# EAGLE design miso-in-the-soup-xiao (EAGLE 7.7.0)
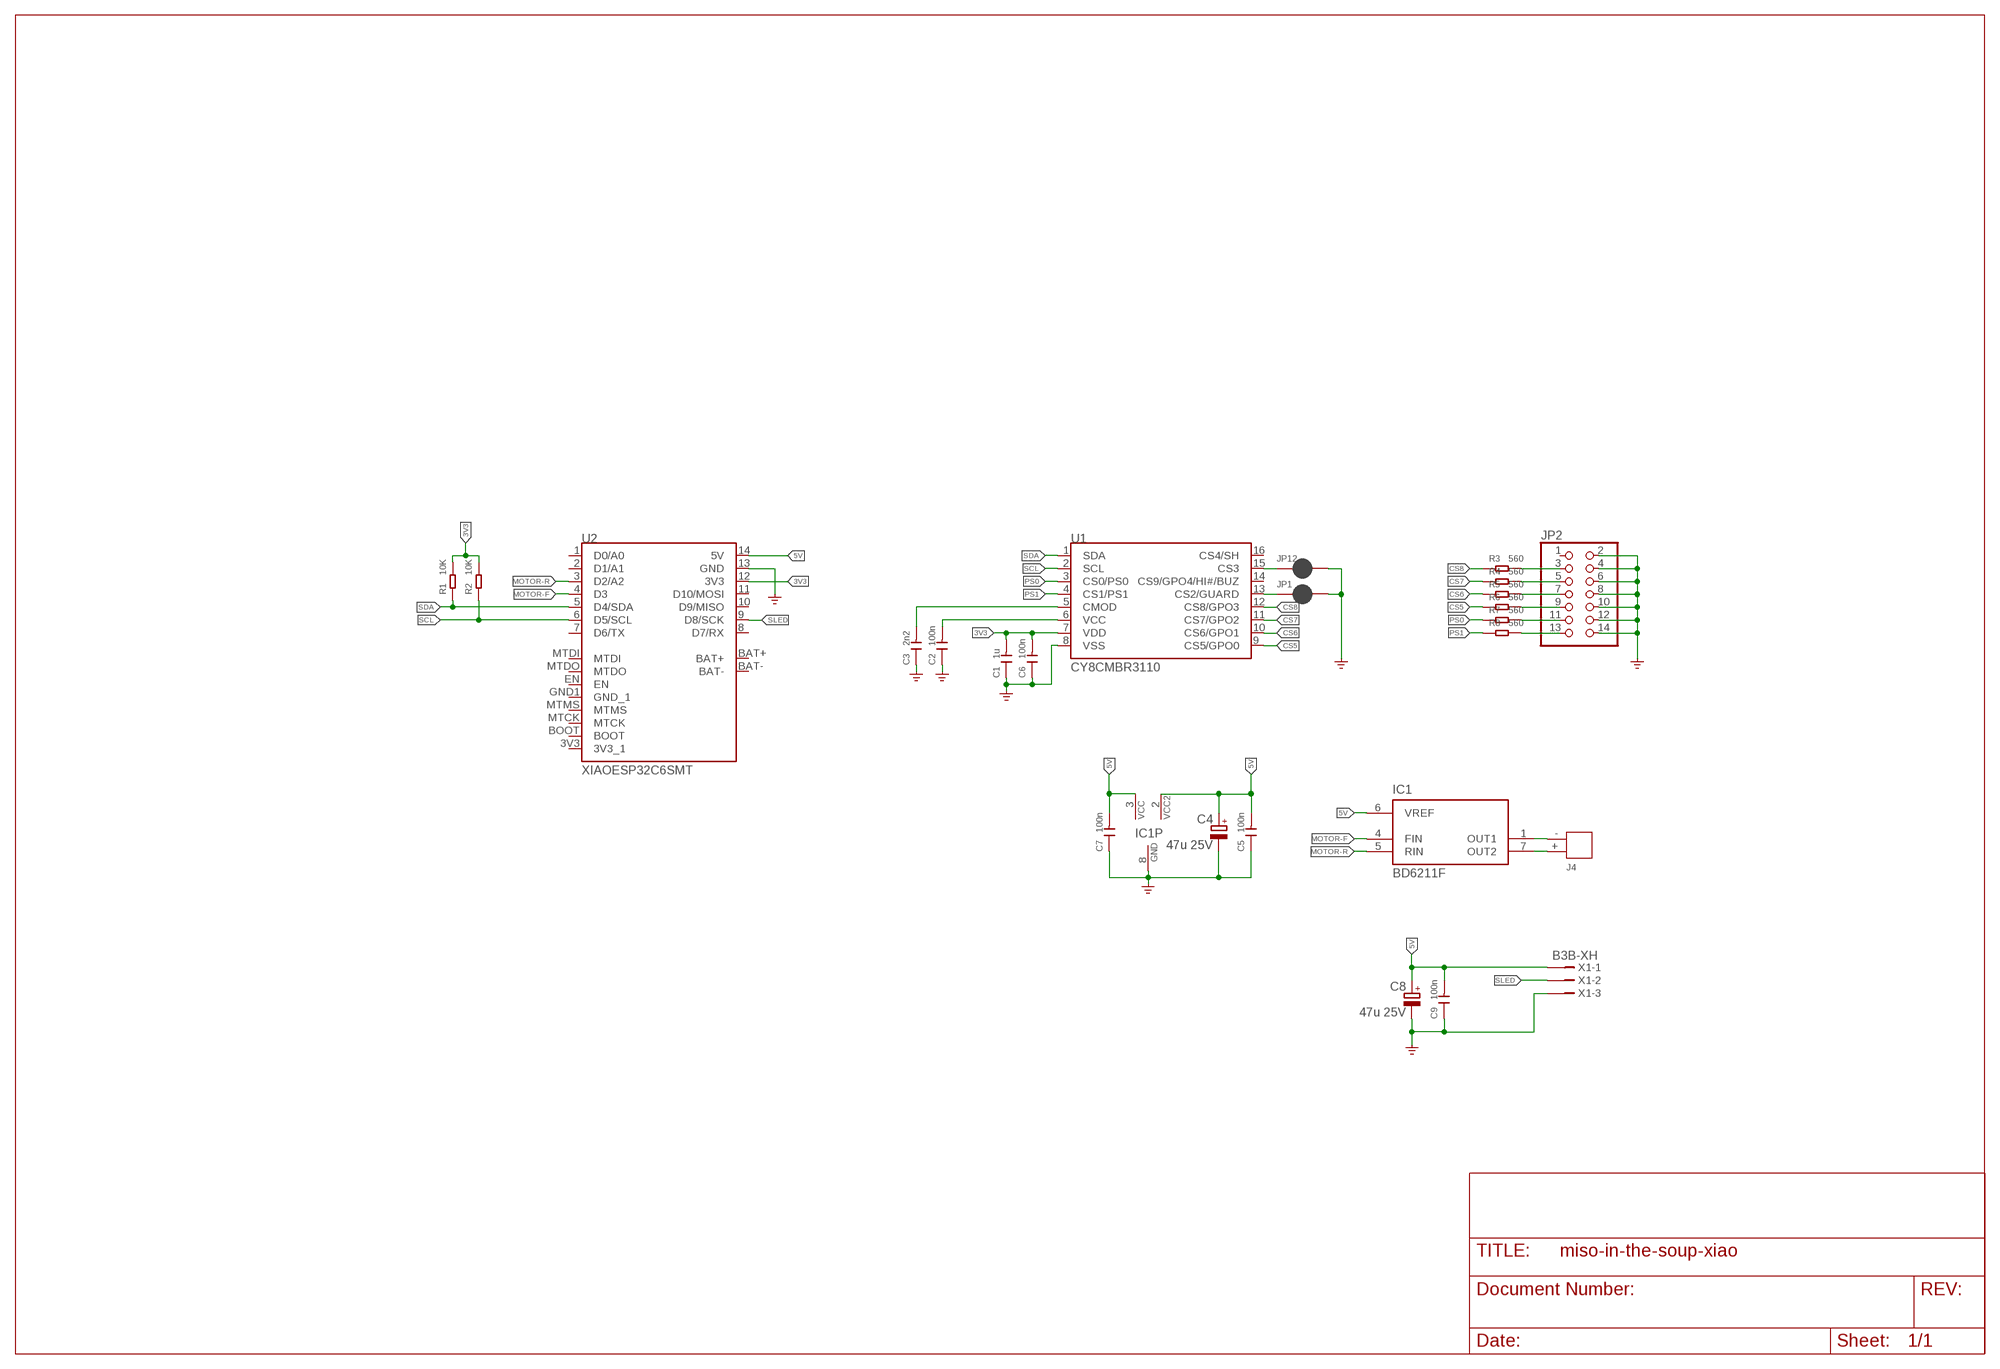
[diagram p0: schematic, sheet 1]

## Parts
C1  1u  C-0603  [C0603]
C2  100n  C-0603  [C0603]
C3  2n2  C-0603  [C0603]
C4  47u 25V  CPOL-EU153CLV-0605  [153CLV-0605]
C5  100n  C-0603  [C0603]
C6  100n  C-0603  [C0603]
C7  100n  C-0603  [C0603]
C8  47u 25V  CPOL-EU153CLV-0605  [153CLV-0605]
C9  100n  C-0603  [C0603]
IC1  BD6211F  [SO08]
J4  JST-2P-DIP'2.0'  [H2-2.0-6X4.5MM]
JP1  JUMPER-SMT_2_NC_PASTE_SILK  [SMT-JUMPER_2_NC_PASTE_SILK]
JP2  PINHD-2X7  [2X07]
JP12  JUMPER-SMT_2_NC_PASTE_SILK  [SMT-JUMPER_2_NC_PASTE_SILK]
R1  10K  R-0603  [R0603]
R2  10K  R-0603  [R0603]
R3  560  R-0603  [R0603]
R4  560  R-0603  [R0603]
R5  560  R-0603  [R0603]
R6  560  R-0603  [R0603]
R7  560  R-0603  [R0603]
R8  560  R-0603  [R0603]
U1  CY8CMBR3110  [SO16]
U2  XIAOESP32C6SMT  [XIAOESP32C6-SMT]
X1  B3B-XH  [B3B-XH]

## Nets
3V3: C1.2 C6.2 R1.2 R2.2 U1.7(VDD) U2.12(3V3)
5V: C4.+ C5.2 C7.2 C8.+ C9.2 IC1.2(VCC2) IC1.3(VCC) IC1.6(VREF) U2.14(5V) X1.1
CS5: R6.1 U1.9(CS5/GPO0)
CS6: R5.1 U1.10(CS6/GPO1)
CS7: R4.1 U1.11(CS7/GPO2)
CS8: R3.1 U1.12(CS8/GPO3)
GND: C1.1 C2.1 C3.1 C4.- C5.1 C6.1 C7.1 C8.- C9.1 IC1.8(GND) JP1.2 JP2.2 JP2.4 JP2.6 JP2.8 JP2.10 JP2.12 JP2.14 JP12.2 U1.8(VSS) U2.13(GND) X1.3 ; supply symbol labelled GND_POWER
MOTOR-F: IC1.4(FIN) U2.4(D3)
MOTOR-R: IC1.5(RIN) U2.3(D2/A2)
N$1: C2.2 U1.6(VCC)
N$2: C3.2 U1.5(CMOD)
N$3: JP12.1 U1.15(CS3)
N$4: JP1.1 U1.13(CS2/GUARD)
N$5: JP2.3 R3.2
N$6: JP2.5 R4.2
N$7: JP2.7 R5.2
N$8: JP2.9 R6.2
N$9: JP2.11 R7.2
N$10: JP2.13 R8.2
N$11: IC1.7(OUT2) J4.+
N$12: IC1.1(OUT1) J4.-
PS0: R7.1 U1.3(CS0/PS0)
PS1: R8.1 U1.4(CS1/PS1)
SCL: R2.1 U1.2(SCL) U2.6(D5/SCL)
SDA: R1.1 U1.1(SDA) U2.5(D4/SDA)
SLED: U2.9(D8/SCK) X1.2
Unconnected: JP2.1 U1.14(CS9/GPO4/HI#/BUZ) U1.16(CS4/SH) U2.1(D0/A0) U2.2(D1/A1) U2.7(D6/TX) U2.8(D7/RX) U2.10(D9/MISO) U2.11(D10/MOSI) U2.BOOT U2.EN U2.MTCK U2.MTDI U2.MTDO U2.MTMS

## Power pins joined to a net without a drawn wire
3V3_1: U2.3V3(3V3_1)
BAT+: U2.BAT+
BAT-: U2.BAT-
GND_1: U2.GND1(GND_1)

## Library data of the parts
C1-C3 C5-C7 C9 = Discrete-small:C*: Ceramic Capacitors
C4 C8 = rcl:CPOL-EU: POLARIZED CAPACITOR, European symbol
IC1 = matsujirushi:BD621*?: ROHM H-BRIDGE DRIVER FOR BRUSH MOTORS
J4 = Connector-new:JST-2P-DIP: 2P-2.0:320110049;2P-2.0-90D:320110027;2P-2.54:320110053;2P-2.54-90D:320110000
JP1 JP12 = SparkFun-Jumpers:JUMPER-SMT_2_NC_PASTE: Normally closed solder jumper
JP2 = pinhead:PINHD-2X7: PIN HEADER
R1-R8 = Discrete-small:R*
U1 = matsujirushi:CY8CMBR3110
U2 = matsujirushi:XIAOESP32C6
X1 = matsujirushi:?3B-XH

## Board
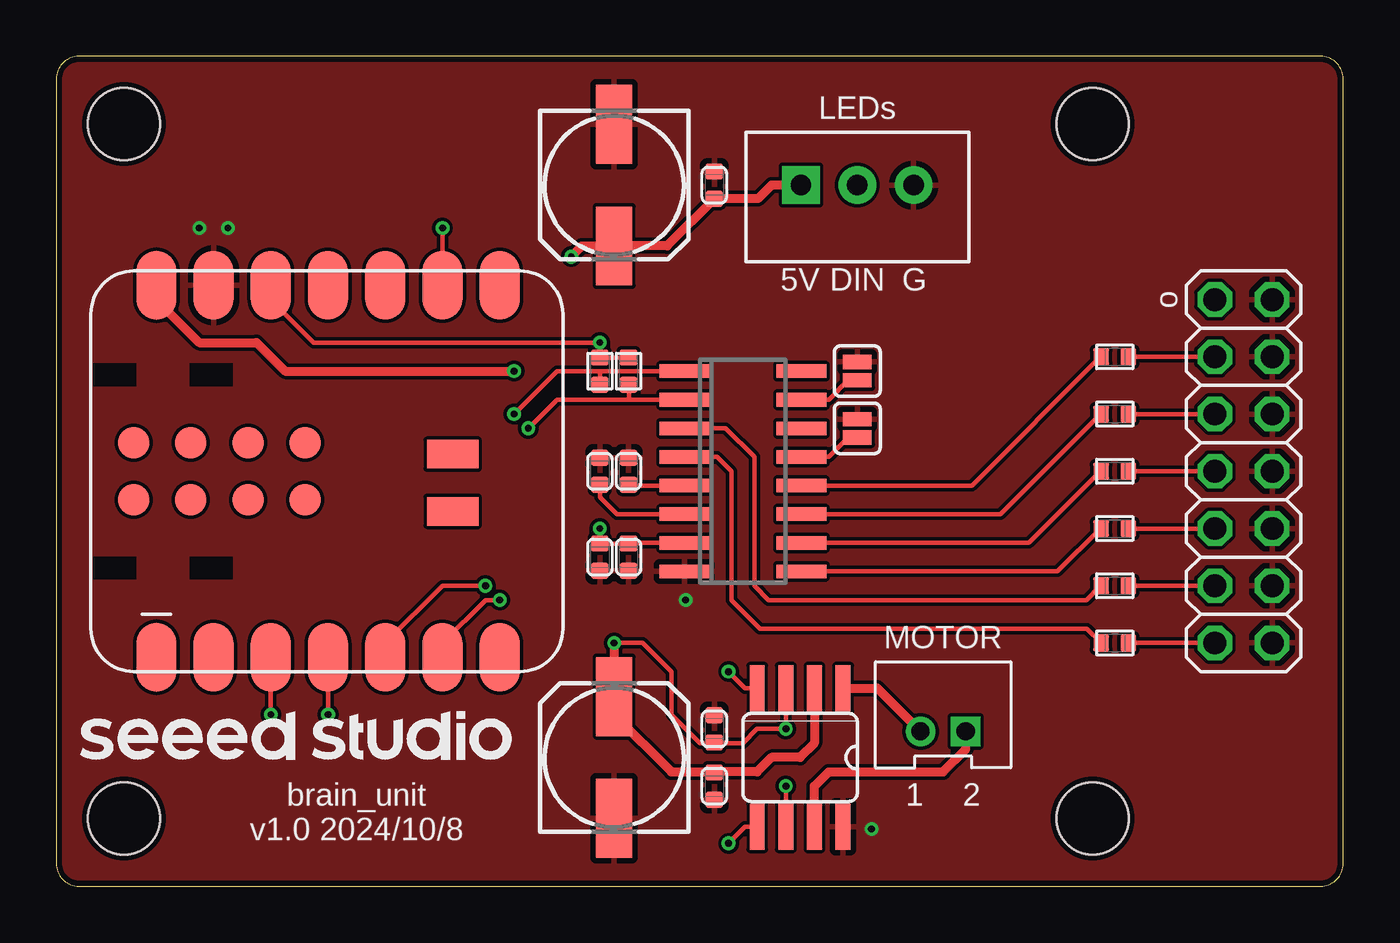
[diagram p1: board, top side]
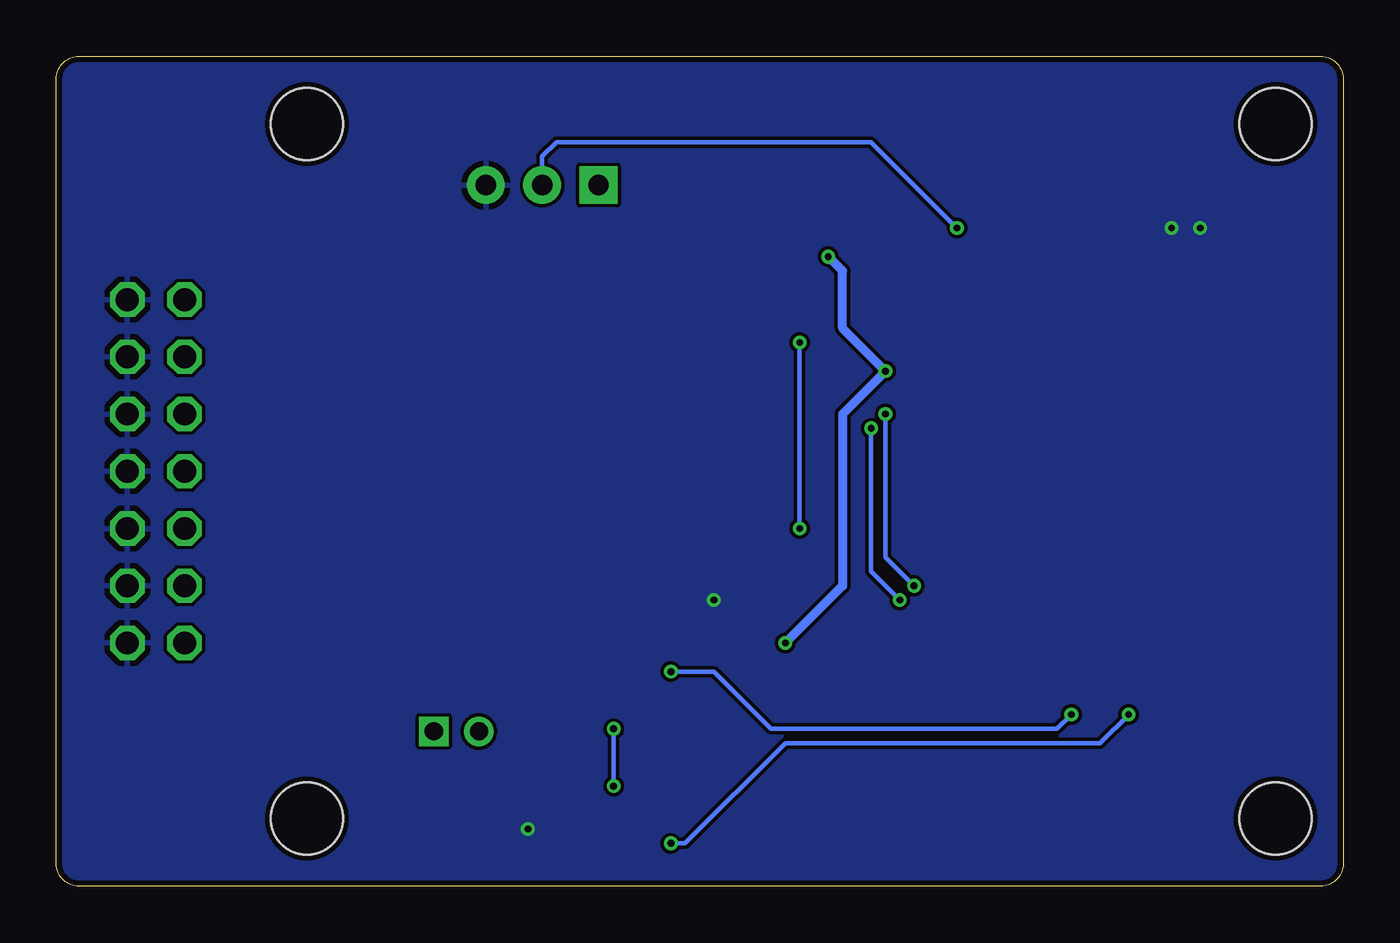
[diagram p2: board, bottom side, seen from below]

Size 57.13 x 36.83 mm. Coordinates in mm from the lower left corner, seen from the top.
Outline: 0,35.83 0,1 arc90 1,0 56.13,0 arc90 57.13,1 57.13,35.83 arc90 56.13,36.83 1,36.83 arc90 0,35.83
Copper layers (1*16): Top 0.035mm / dielectric 1.5mm / Bottom 0.035mm
Design rules "SeeedStudio_2layer_DRU_no_angle_20140221": minimum track width 6mil, minimum drill 12mil, track to track 6mil, track to pad 6mil, pad to pad 6mil, via to via 6mil, smd to smd 0mil, copper to edge 10mil, drill to drill 10mil, minimum pad ring 10mil, minimum via ring 6mil, stop-mask expansion 2mil, vias tented up to drill 100mil, thermal gap 10mil
Holes 3.2 mm at 3,3 3,33.83 46,33.83 46,3

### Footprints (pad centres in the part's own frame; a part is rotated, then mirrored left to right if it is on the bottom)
C0603 = smd 0.762 x 0.696: 1 0,0.602; 2 0,-0.602
153CLV-0605 = smd 3.5 x 1.6: + 2.7,0; - -2.7,0
SO08 = smd 0.66 x 2.032: 1 -1.905,-3.073; 2 -0.635,-3.073; 3 0.635,-3.073; 4 1.905,-3.073; 5 1.905,3.073; 6 0.635,3.073; 7 -0.635,3.073; 8 -1.905,3.073
H2-2.0-6X4.5MM = drill 0.8 pad 1.3 square: + -1,0.75 | drill 0.8 pad 1.3: - 1,0.75
SMT-JUMPER_2_NC_PASTE_SILK = smd 0.635 x 1.27: 1 -0.406,0; 2 0.406,0
2X07 = drill 1.016 octagon: 1 -7.62,-1.27; 2 -7.62,1.27; 3 -5.08,-1.27; 4 -5.08,1.27; 5 -2.54,-1.27; 6 -2.54,1.27; 7 0,-1.27; 8 0,1.27; 9 2.54,-1.27; 10 2.54,1.27; 11 5.08,-1.27; 12 5.08,1.27; 13 7.62,-1.27; 14 7.62,1.27
R0603 = smd 0.762 x 0.696: 1 0,0.602; 2 0,-0.602
SO16 = smd 0.6 x 2.2: 1 -4.445,-2.6; 2 -3.175,-2.6; 3 -1.905,-2.6; 4 -0.635,-2.6; 5 0.635,-2.6; 6 1.905,-2.6; 7 3.175,-2.6; 8 4.445,-2.6; 9 4.445,2.6; 10 3.175,2.6; 11 1.905,2.6; 12 0.635,2.6; 13 -0.635,2.6; 14 -1.905,2.6; 15 -3.175,2.6; 16 -4.445,2.6
XIAOESP32C6-SMT = smd 1.778 x 3.048: 1 7.62,8.255; 2 5.08,8.255; 3 2.54,8.255; 4 0,8.255; 5 -2.54,8.255; 6 -5.08,8.255; 7 -7.62,8.255; 8 -7.62,-8.255; 9 -5.08,-8.255; 10 -2.54,-8.255; 11 0,-8.255; 12 2.54,-8.255; 13 5.08,-8.255; 14 7.62,-8.255 | smd 1.397 x 1.397: 3V3 1.016,-1.27; BOOT 1.016,1.27; EN 6.096,1.27; GND1 6.096,-1.27; MTCK 3.556,-1.27; MTDI 8.636,1.27; MTDO 8.636,-1.27; MTMS 3.556,1.27 | smd 2.286 x 1.27: BAT+ -5.537,1.778; BAT- -5.537,-0.762
B3B-XH = drill 0.9 pad 1.676 square: 1 2.5,0 | drill 0.9 pad 1.676: 2 0,0; 3 -2.5,0

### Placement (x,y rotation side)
C1  24.13,14.61 180 top
C2  24.13,18.41 0 top
C3  25.4,18.41 0 top
C4  24.77,5.71 90 top
C5  29.21,4.45 180 top
C6  25.4,14.61 180 top
C7  29.21,6.99 0 top
C8  24.77,31.11 270 top
C9  29.21,31.11 0 top
IC1  33.02,5.71 180 top
J4  39.37,7.62 180 top
JP1  35.56,20.32 90 top
JP2  52.7,18.41 270 top
JP12  35.56,22.86 90 top
R1  24.13,22.86 180 top
R2  25.4,22.86 180 top
R3  46.99,23.5 90 top
R4  46.99,20.95 90 top
R5  46.99,18.41 90 top
R6  46.99,15.88 90 top
R7  46.99,13.34 90 top
R8  46.99,10.79 90 top
U1  30.48,18.41 270 top
U2  12.06,18.41 180 top
X1  35.56,31.11 180 top

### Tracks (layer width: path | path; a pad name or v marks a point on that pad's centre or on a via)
3V3  (via drill 0.3)
  Top 0.203: U1.7 25.4,15.24 C6.2 C1.2 v24.13,15.88 | R2.2 R1.2 v24.13,24.13 11.43,24.13 9.53,26.04 U2.12
  Bottom 0.203: v24.13,15.88 v24.13,24.13
5V  (via drill 0.3)
  Top 0.203: IC1.3 v32.38,6.99 31.11,6.99 30.48,6.35 29.21,6.35 | 29.21,6.35 28.57,6.35 27.3,7.62 27.3,9.53 26.04,10.79 v24.77,10.79 | 29.21,6.35 C7.2 | IC1.6 v32.38,4.45 | U2.14 4.45,26.04
  Top 0.406: IC1.2 33.66,6.35 33.02,5.71 31.75,5.71 31.11,5.08 29.21,5.08 | v24.77,10.79 C4.+ 24.77,7.62 27.3,5.08 29.21,5.08 | 4.45,26.04 6.35,24.13 8.89,24.13 10.16,22.86 v20.32,22.86 | 29.21,5.08 C5.2 | v22.86,27.94 23.34,28.41 C8.+ 27.11,28.41 C9.2 31.15,30.51 31.75,31.11 X1.1
  Bottom 0.203: v32.38,4.45 v32.38,6.99
  Bottom 0.406: v24.77,10.79 22.23,13.34 22.23,20.95 v20.32,22.86 22.23,24.77 22.23,27.3 v22.86,27.94
CS5
  Top 0.203: U1.9 44.45,13.97 46.35,15.88 R6.1
CS6
  Top 0.203: U1.10 43.18,15.24 46.35,18.41 R5.1
CS7
  Top 0.203: U1.11 41.91,16.51 46.35,20.95 R4.1
CS8
  Top 0.203: U1.12 40.64,17.78 46.35,23.5 R3.1
GND  (via drill 0.3)
  other vias: 6.35,29.21 7.62,29.21 36.2,2.54 27.94,12.7
  pour Top: 0,36.83 57.15,36.83 57.15,0 0,0
  pour Bottom: 0,36.83 57.15,36.83 57.15,0 0,0
MOTOR-F  (via drill 0.3)
  Top 0.203: IC1.4 30.58,8.79 v29.84,9.53 | v12.06,7.62 U2.4
  Bottom 0.203: v29.84,9.53 27.94,9.53 25.4,6.99 12.7,6.99 v12.06,7.62
MOTOR-R  (via drill 0.3)
  Top 0.203: IC1.5 30.58,2.64 v29.84,1.91 | v9.53,7.62 U2.3
  Bottom 0.203: v9.53,7.62 10.79,6.35 24.77,6.35 29.21,1.91 v29.84,1.91
N$1
  Top 0.203: U1.6 24.89,16.51 24.13,17.27 C2.2
N$2
  Top 0.203: U1.5 25.4,17.78 C3.2
N$3
  Top 0.203: JP12.1 35.15,22.45 34.29,21.59 U1.15
N$4
  Top 0.203: JP1.1 35.15,19.91 34.29,19.05 U1.13
N$5
  Top 0.203: R3.2 JP2.3
N$6
  Top 0.203: JP2.5 R4.2
N$7
  Top 0.203: JP2.7 R5.2
N$8
  Top 0.203: JP2.9 R6.2
N$9
  Top 0.203: JP2.11 R7.2
N$10
  Top 0.203: JP2.13 R8.2
N$11
  Top 0.406: IC1.7 33.66,4.45 34.29,5.08 39.37,5.08 40.37,6.08 J4.+
N$12
  Top 0.406: IC1.1 36.45,8.79 J4.-
PS0
  Top 0.203: U1.3 29.72,20.32 30.99,19.05 30.99,13.34 31.62,12.7 45.72,12.7 46.35,13.34 R7.1
PS1
  Top 0.203: U1.4 29.34,19.05 29.97,18.41 29.97,12.7 31.24,11.43 45.75,11.43 R8.1
SCL  (via drill 0.3)
  Top 0.203: R2.1 25.43,21.59 | 25.43,21.59 U1.2 | 25.43,21.59 22.23,21.59 v20.95,20.32 | v19.68,12.7 19.05,12.7 17.14,10.79 U2.6
  Bottom 0.203: v20.95,20.32 20.95,13.97 v19.68,12.7
SDA  (via drill 0.3)
  Top 0.203: 14.61,9.53 U2.5 14.61,10.79 17.14,13.34 v19.05,13.34 | v20.32,20.95 22.23,22.86 24.13,22.86 | 24.13,22.86 U1.1 | R1.1 24.13,22.86
  Bottom 0.203: v19.05,13.34 20.32,14.61 v20.32,20.95
SLED  (via drill 0.3)
  Top 0.203: U2.9 v17.14,29.21
  Bottom 0.203: v17.14,29.21 20.95,33.02 34.92,33.02 35.56,32.38 X1.2

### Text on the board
tPlace: LEDs | 5V | DIN | G | o | MOTOR | 1 | 2 | brain_unit / v1.0 2024/10/8

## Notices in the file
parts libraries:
SparkFun-Jumpers: Licensing: Creative Commons ShareAlike 4.0 International - https://creativecommons.org/licenses/by-sa/4.0
